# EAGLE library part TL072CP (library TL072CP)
TL072 Dual Low-Noise JFET-Input General-Purpose Operational Amplifier Source: Datasheet
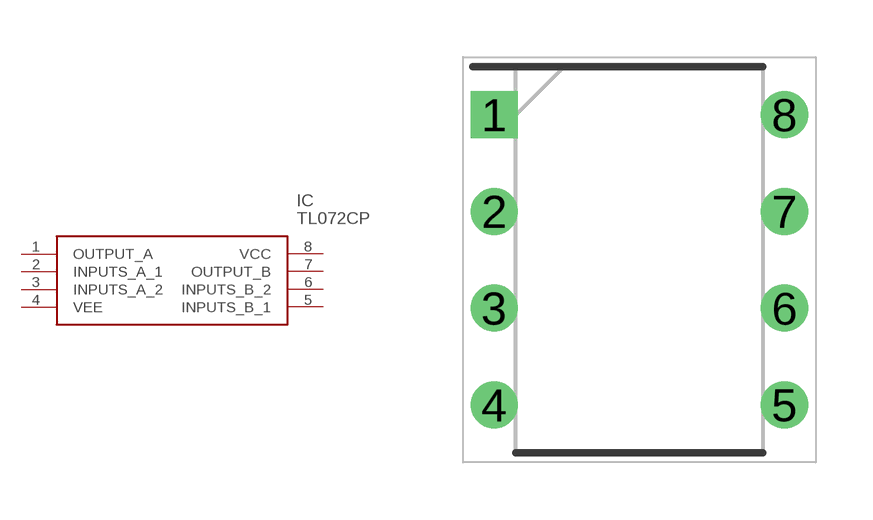
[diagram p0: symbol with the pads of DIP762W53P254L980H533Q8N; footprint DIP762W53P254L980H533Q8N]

Designator prefix IC

## TL072CP (Description: TL072 Dual Low-Noise JFET-Input General-Purpose Operational Amplifier; Height: 5.33mm; Manufacturer_Name: onsemi; Manufacturer_Part_Number: TL072CP; Mouser_Part_Number: N/A; Mouser_Price-Stock: https://www.mouser.co.uk/ProductDetail/onsemi/TL072CP?qs=PJJcWtbOkNWgH%2F5P%252B5rz0g%3D%3D)  [DIP762W53P254L980H533Q8N]
1  OUTPUT_A
2  INPUTS_A_1
3  INPUTS_A_2
4  VEE
5  INPUTS_B_1
6  INPUTS_B_2
7  OUTPUT_B
8  VCC

## Footprint DIP762W53P254L980H533Q8N (pad centres in mm)
8-DIP
drill 0.73 pad 1.13 square: 1 -3.81,3.81
drill 0.73 pad 1.13: 2 -3.81,1.27; 3 -3.81,-1.27; 4 -3.81,-3.81; 5 3.81,-3.81; 6 3.81,-1.27; 7 3.81,1.27; 8 3.81,3.81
